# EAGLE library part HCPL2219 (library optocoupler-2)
HEWLETT PACKARD OPTO COUPLER
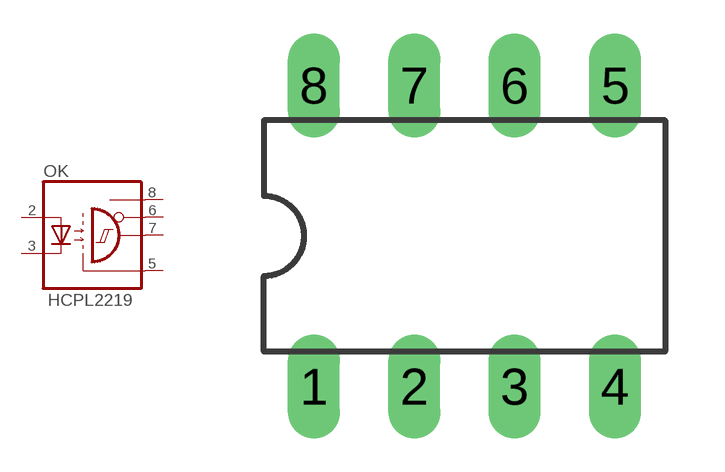
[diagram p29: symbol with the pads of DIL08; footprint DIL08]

Designator prefix OK

## HCPL2219  [DIL08]
2  A  pas
3  C  pas
5  GND  pas
6  VE  pas
7  VO  pas
8  VCC  pas

## Footprint DIL08 (pad centres in mm)
Dual In Line Package
drill 0.813 long: 1 -3.81,-3.81; 2 -1.27,-3.81; 3 1.27,-3.81; 4 3.81,-3.81; 5 3.81,3.81; 6 1.27,3.81; 7 -1.27,3.81; 8 -3.81,3.81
